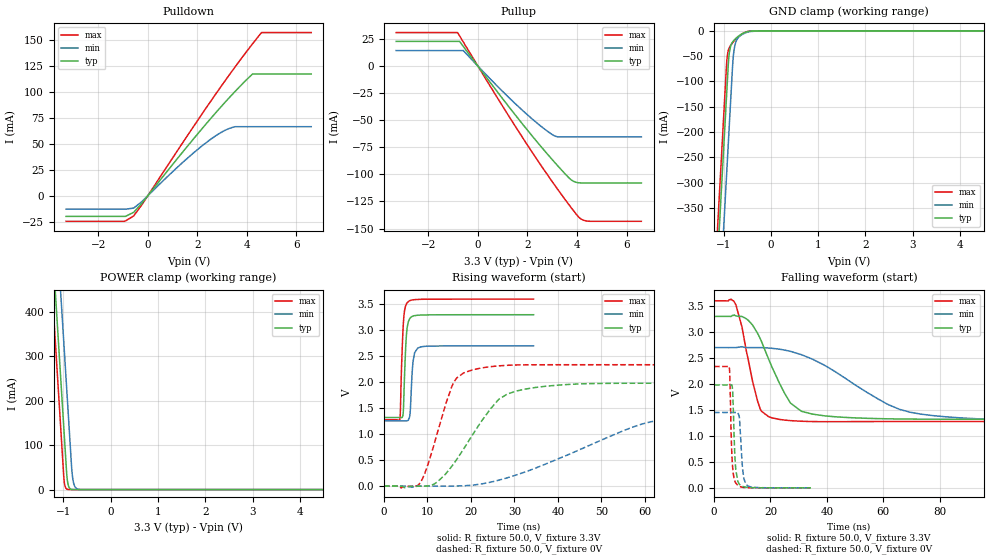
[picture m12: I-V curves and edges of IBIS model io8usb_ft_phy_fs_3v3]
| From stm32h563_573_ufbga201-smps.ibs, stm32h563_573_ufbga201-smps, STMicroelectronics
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[Model]   io8usb_ft_phy_fs_3v3
Model_type I/O
Polarity   Non-Inverting
Enable   Active-Low
| CAP_THRESHOLD on pad DPFT is "UDTCAPC" :
| Rising=20.0% of vddiom   Falling=80.0% of vddiom
| C_comp min and max val. don't necessarily correlate with the min and max pvt
| but are the smallest and greatest pad capacitance found.
| var   typ   min   max
C_comp   8.88570pF  8.80266pF  8.92058pF
|C_comp_pullup   6.10735pF  5.78805pF  5.62765pF
|C_comp_pulldown   2.77835pF  3.01461pF  3.29293pF
Vinl = 1.35V
Vinh = 1.8V
Vmeas = 1.65V   | Reference voltage for timing measurements
Cref  = 50.0pF   | Timing specification test load capacitance value
Rref  = 1.0MOhm   | Timing specification test load resistance value
Vref  = 1.815V   | Timing specification test load voltage
[Model Spec]
| TIME_THRESHOLD on pin ZIUSBPV11 is "CMOS" :
| Rising=40.0% of vdd   Falling=60.0% of vdd
Vinl 1.31380V 1.08880V 1.42380V
Vinh 1.79320V 1.51020V 1.91620V
| variable   typ   min   max
[Temperature Range] 25.0 125.0 -40.0
| variable   typ   min   max
[Voltage Range] 3.3V 2.7V 3.6V
| variable   typ   min   max
[POWER Clamp Reference] 3.3V 2.7V 3.6V
| variable   typ   min   max
[GND Clamp Reference] 0V 0V 0V
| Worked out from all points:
|   slope of the pulldown table from 0 to 0.495 V, typ, clamps not added: 33.1 ohm
|   slope of the pullup table from 0 to 0.495 V, typ, clamps not added: 32.9 ohm
|   GND clamp passes 1 mA (typ) near -0.46 V on its own axis
|   POWER clamp passes 1 mA (typ) near -0.84 V on its own axis
|   rising waveform, R_fixture 50.0, V_fixture 3.3V: 20-80 % time 589ps typ, 600ps min, 595ps max; typ from 1.32 V to 3.3 V
|   falling waveform, R_fixture 50.0, V_fixture 3.3V: 20-80 % time 10.1ns typ, 26.9ns min, 5.39ns max; typ from 3.3 V to 1.32 V
|   rising waveform, R_fixture 50.0, V_fixture 0V: 20-80 % time 9.77ns typ, 24.9ns min, 5.09ns max; typ from 0 V to 1.98 V
|   falling waveform, R_fixture 50.0, V_fixture 0V: 20-80 % time 860ps typ, 1.08ns min, 778ps max; typ from 1.98 V to 0 V
[POWER Clamp]
-3.3V     4.068A     4.259A     3.957A
-1.25V    582.8mA    774.2mA    471.5mA
-1.16V    429.8mA    621.2mA    318.5mA
-1.05V    242.8mA    434.2mA    131.5mA
-980mV    123.8mA    315.2mA    17.95mA
-960mV    89.81mA    281.2mA    6.634mA
-920mV    26.3mA     213.2mA    906uA
-880mV    5.543mA    145.2mA    123.7uA
-810mV    363.5uA    33.6mA     3.798uA
-770mV    76.63uA    10.47mA    519.9nA
-690mV    3.411uA    1.017mA    10.89nA
6.6V      0A         0A         0A
[GND Clamp]
-3.3V     -4.147A    -4.304A    -4.084A
-1.25V    -662.3mA   -818.9mA   -599mA
-940mV    -135.3mA   -291.9mA   -71.97mA
-910mV    -84.3mA    -240.9mA   -43.19mA
-890mV    -54.53mA   -206.9mA   -36.04mA
-870mV    -38.95mA   -172.9mA   -31.83mA
-810mV    -22.29mA   -70.86mA   -23.78mA
-780mV    -18.66mA   -39.68mA   -20.49mA
-750mV    -15.77mA   -25.18mA   -17.46mA
-710mV    -12.47mA   -16.15mA   -13.75mA
-540mV    -3.025mA   -4.157mA   -2.753mA
6.6V      24.07nA    4.253uA    975.9pA
| variable   typ   min   max
[Pullup Reference] 3.3V 2.7V 3.6V
| variable   typ   min   max
[Pulldown Reference] 0V 0V 0V
[Pullup]
-3.3V     22.83mA    14.39mA    31mA
-820mV    22.83mA    14.39mA    31mA
-740mV    22.83mA    14.39mA    27.95mA
-590mV    18.16mA    14.39mA    22.24mA
1.32V     -39.61mA   -30.57mA   -48.77mA
2.85V     -82.4mA    -60.84mA   -101.8mA
3.19V     -91.23mA   -65.16mA   -112.8mA
3.7V      -103.7mA   -65.39mA   -128.7mA
4.06V     -107.7mA   -65.39mA   -139.2mA
4.22V     -107.9mA   -65.39mA   -141.9mA
4.51V     -107.9mA   -65.39mA   -143.3mA
6.6V      -107.9mA   -65.39mA   -143.3mA
[Pulldown]
-3.3V     -19.88mA   -12.95mA   -24.65mA
-940mV    -19.88mA   -12.95mA   -24.65mA
-570mV    -15.96mA   -11.9mA    -19.44mA
-220mV    -6.69mA    -5.247mA   -8.037mA
1.48V     44.27mA    33.69mA    53.76mA
2.17V     64.17mA    47.77mA    78.28mA
2.8V      81.66mA    58.79mA    100.1mA
3.19V     92.07mA    63.96mA    113.3mA
3.51V     100.3mA    66.56mA    123.9mA
4.23V     117.5mA    66.66mA    146.6mA
4.59V     117.5mA    66.66mA    157.5mA
6.6V      117.5mA    66.66mA    157.5mA
[Ramp]
dV/dt_r 1.18821V/9.67362ns 866.70792mV/24.84354ns 1.40193V/5.07203ns
dV/dt_f 1.18779V/10.0041ns 865.50298mV/26.67598ns 1.3938V/5.29566ns
R_load = 50.0
| Removed startup time: 0s 0s 0s  .
| Removed end time: 34.4ns.
[Rising Waveform]
R_fixture   = 50.0
V_fixture   = 3.3V
V_fixture_min = 2.7V
V_fixture_max = 3.6V
0s        1.32V      1.257V     1.277V
3.65ns    1.32V      1.257V     1.288V
3.75ns    1.32V      1.257V     1.376V
4.5ns     1.521V     1.257V     3.181V
5.05ns    2.754V     1.257V     3.486V
5.6ns     3.163V     1.268V     3.553V
6ns       3.232V     1.396V     3.573V
6.7ns     3.275V     2.404V     3.587V
7.75ns    3.29V      2.656V     3.594V
34.4ns    3.3V       2.7V       3.6V
| Removed startup time: 0s 0s 0s  .
| Removed end time: 189.4ns.
[Falling Waveform]
R_fixture   = 50.0
V_fixture   = 3.3V
V_fixture_min = 2.7V
V_fixture_max = 3.6V
0s        3.3V       2.7V       3.6V
7.75ns    3.307V     2.7V       3.522V
12ns      3.231V     2.699V     2.498V
15.45ns   2.973V     2.7V       1.665V
20.55ns   2.323V     2.686V     1.347V
27.05ns   1.634V     2.628V     1.294V
39.4ns    1.385V     2.351V     1.274V
61.85ns   1.329V     1.601V     1.277V
73.45ns   1.323V     1.418V     1.277V
189.4ns   1.32V      1.257V     1.277V
| Removed startup time: 0s 0s 0s  .
| Removed end time: 99.4ns.
[Rising Waveform]
R_fixture   = 50.0
V_fixture   = 0V
V_fixture_min = 0V
V_fixture_max = 0V
0s        24.82nV    1.065uV    39.76nV
8.2ns     -1.838mV   -1.542mV   47.72mV
10.2ns    2.709mV    -684.9uV   435.6mV
12.2ns    73.26mV    -674uV     1.001V
15.8ns    403.2mV    165.2uV    1.953V
20.3ns    978.4mV    16.48mV    2.237V
26.4ns    1.671V     113.2mV    2.315V
34.5ns    1.895V     334.7mV    2.336V
62.9ns    1.98V      1.264V     2.337V
99.4ns    1.98V      1.445V     2.337V
| Removed startup time: 0s 0s 0s  .
| Removed end time: 34.35ns.
[Falling Waveform]
R_fixture   = 50.0
V_fixture   = 0V
V_fixture_min = 0V
V_fixture_max = 0V
0s        1.98V      1.451V     2.337V
5.35ns    1.98V      1.451V     2.329V
5.6ns     1.98V      1.451V     2.125V
6.05ns    1.981V     1.451V     1.052V
6.4ns     1.958V     1.451V     546.4mV
7.7ns     352.2mV    1.451V     91.95mV
8.9ns     74.21mV    1.381V     33.24mV
10.1ns    29.35mV    365.7mV    10.98mV
11.25ns   14.26mV    73.13mV    3.146mV
34.35ns   162.6uV    421.2uV    147.6uV
